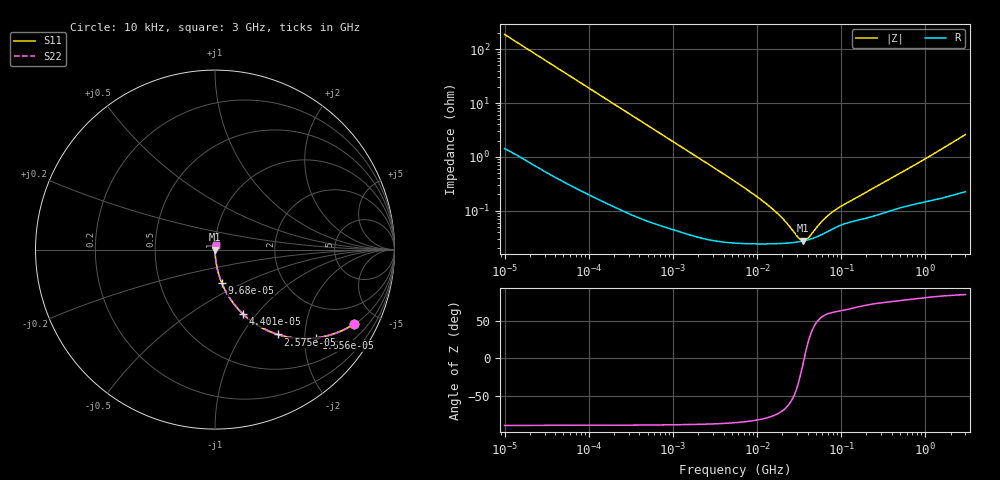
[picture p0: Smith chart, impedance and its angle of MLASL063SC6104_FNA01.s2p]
! MLASL063SC6104_FNA01  S-PARAMETER MODEL  ( Standard Model )
! Model Generated by TAIYO YUDEN Corporation (http://www.ty-top.com)
! Version 1.0
! TAIYO YUDEN Control No. 220601
! Copyright(c) 2013 TAIYO YUDEN CO.,LTD. All Rights Reserved.
! Product Description (link to TY-COMPAS)
! https://ds.yuden.co.jp/TYCOMPAS/or/detail?pn=MLASL063SC6104KFNA01&u=M
! Products Name : Multilayer Ceramic Capacitors
! Characteristics :
!  Capacitance : 0.1 [uF] , Rated Voltage : 10 [V] , TCC : X6S
!  Case Size : 0.6 x 0.3 / 0.024 x 0.012 [mm/inch] , Thickness : 0.3 / 0.012 [mm/inch]
!  (Conditions: Temperature = 25 [degC] , DC Bias Voltage = 0 [V])
! External Node Assignments :
!  1  o---| |---o  2
! GND o---------o GND
! Frequency Range : 10kHz  -  3GHz  [ 401 STEP ]
# MHZ S RI R 50
! Freq[MHz].  S11 Real  S11 Imag  S21 Real  S21 Imag  S12 Real  S12 Imag  S22 Real  S22 Imag
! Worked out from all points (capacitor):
!   401 points, 10 kHz to 3 GHz, reference 50 ohm
!   read as one part in series: C = 84.7 nF near 10.65 kHz
!   lowest |Z| = 27.5 mohm at 35.19 MHz (marker M1)
!   series resonance near 36.45 MHz, so ESL is about 230 pH
!   S11 on the Smith chart (normalised r, x): 10 kHz: 1.03, -3.75; 16.56 kHz: 1.02, -2.27; 25.75 kHz: 1.01, -1.46; 44.01 kHz: 1.01, -0.86; 96.8 kHz: 1.00, -0.39; 3 GHz: 1.00, +0.05
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0.01  0.7769 -0.4126  0.2231 0.4126  0.2231 0.4126  0.7769 -0.4126
0.012083  0.7057 -0.4518  0.2943 0.4518  0.2943 0.4518  0.7057 -0.4518
0.016561  0.5628 -0.492  0.4372 0.492  0.4372 0.492  0.5628 -0.492
0.02575  0.3502 -0.4729  0.6498 0.4729  0.6498 0.4729  0.3502 -0.4729
0.044011  0.158 -0.3603  0.842 0.3603  0.842 0.3603  0.158 -0.3603
0.058452  0.0971 -0.2915  0.9029 0.2915  0.9029 0.2915  0.0971 -0.2915
0.082683  0.0519 -0.217  0.9481 0.217  0.9481 0.217  0.0519 -0.217
0.096801  0.0388 -0.1881  0.9612 0.1881  0.9612 0.1881  0.0388 -0.1881
0.226771  0.00808 -0.0834  0.9919 0.0834  0.9919 0.0834  0.00808 -0.0834
0.683653  0.00133 -0.0281  0.9987 0.0281  0.9987 0.0281  0.00133 -0.0281
5.477226  0.000262 -0.00348  0.9997 0.00348  0.9997 0.00348  0.000262 -0.00348
9.97066  0.000245 -0.00181  0.9998 0.00181  0.9998 0.00181  0.000245 -0.00181
15.50326  0.000244 -0.00103  0.9998 0.00103  0.9998 0.00103  0.000244 -0.00103
21.24962  0.000248 -0.000606  0.9998 0.000606  0.9998 0.000606  0.000248 -0.000606
31.02164  0.000263 -0.000173  0.9997 0.000173  0.9997 0.000173  0.000263 -0.000173
35.19136  0.000273 -3.75e-05  0.9997 3.75e-05  0.9997 3.75e-05  0.000273 -3.75e-05
38.68249  0.000282 6.34e-05  0.9997 -6.34e-05  0.9997 -6.34e-05  0.000282 6.34e-05
45.28751  0.000303 0.000232  0.9997 -0.000232  0.9997 -0.000232  0.000303 0.000232
62.07353  0.000375 0.000572  0.9996 -0.000572  0.9996 -0.000572  0.000375 0.000572
85.08137  0.000485 0.000909  0.9995 -0.000909  0.9995 -0.000909  0.000485 0.000909
374.4521  0.000992 0.00372  0.999 -0.00372  0.999 -0.00372  0.000992 0.00372
3000  0.00291 0.0257  0.9971 -0.0257  0.9971 -0.0257  0.00291 0.0257
